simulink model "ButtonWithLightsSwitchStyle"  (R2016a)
settings: Solver=FixedStepAuto  StartTime=0.0  StopTime=inf  RelTol=1e-3
libraries: miniQ x2

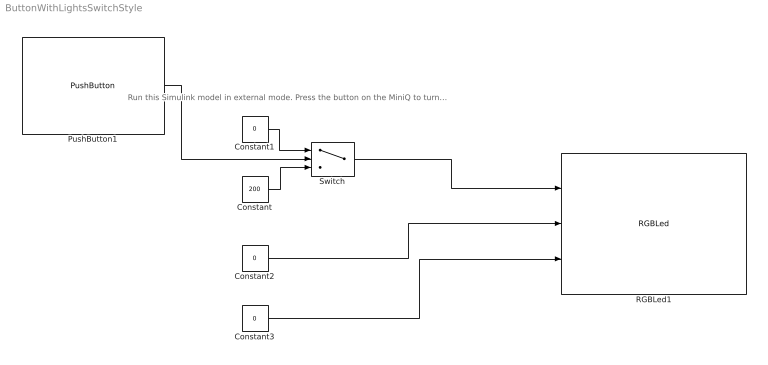
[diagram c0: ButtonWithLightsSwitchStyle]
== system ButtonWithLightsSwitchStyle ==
  note: Run this Simulink model in external mode. Press the button on the MiniQ to turn the red light on or off. This is the result of the switch changing between Constant (200) and Constant1 (0).
  Constant : Constant  Value=200
  Constant1 : Constant  Value=0
  Constant2 : Constant  Value=0
  Constant3 : Constant  Value=0
  PushButton1 : miniQ/PushButton  sampleTime_dd=0.1  debug_dd=off
  RGBLed1 : miniQ/RGBLed
  Switch : Switch  Criteria=u2 > Threshold
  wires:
  PushButton1/1 -> Switch/2
  Constant/1 -> Switch/3
  Constant1/1 -> Switch/1
  Constant2/1 -> RGBLed1/2
  Constant3/1 -> RGBLed1/3
  Switch/1 -> RGBLed1/1
